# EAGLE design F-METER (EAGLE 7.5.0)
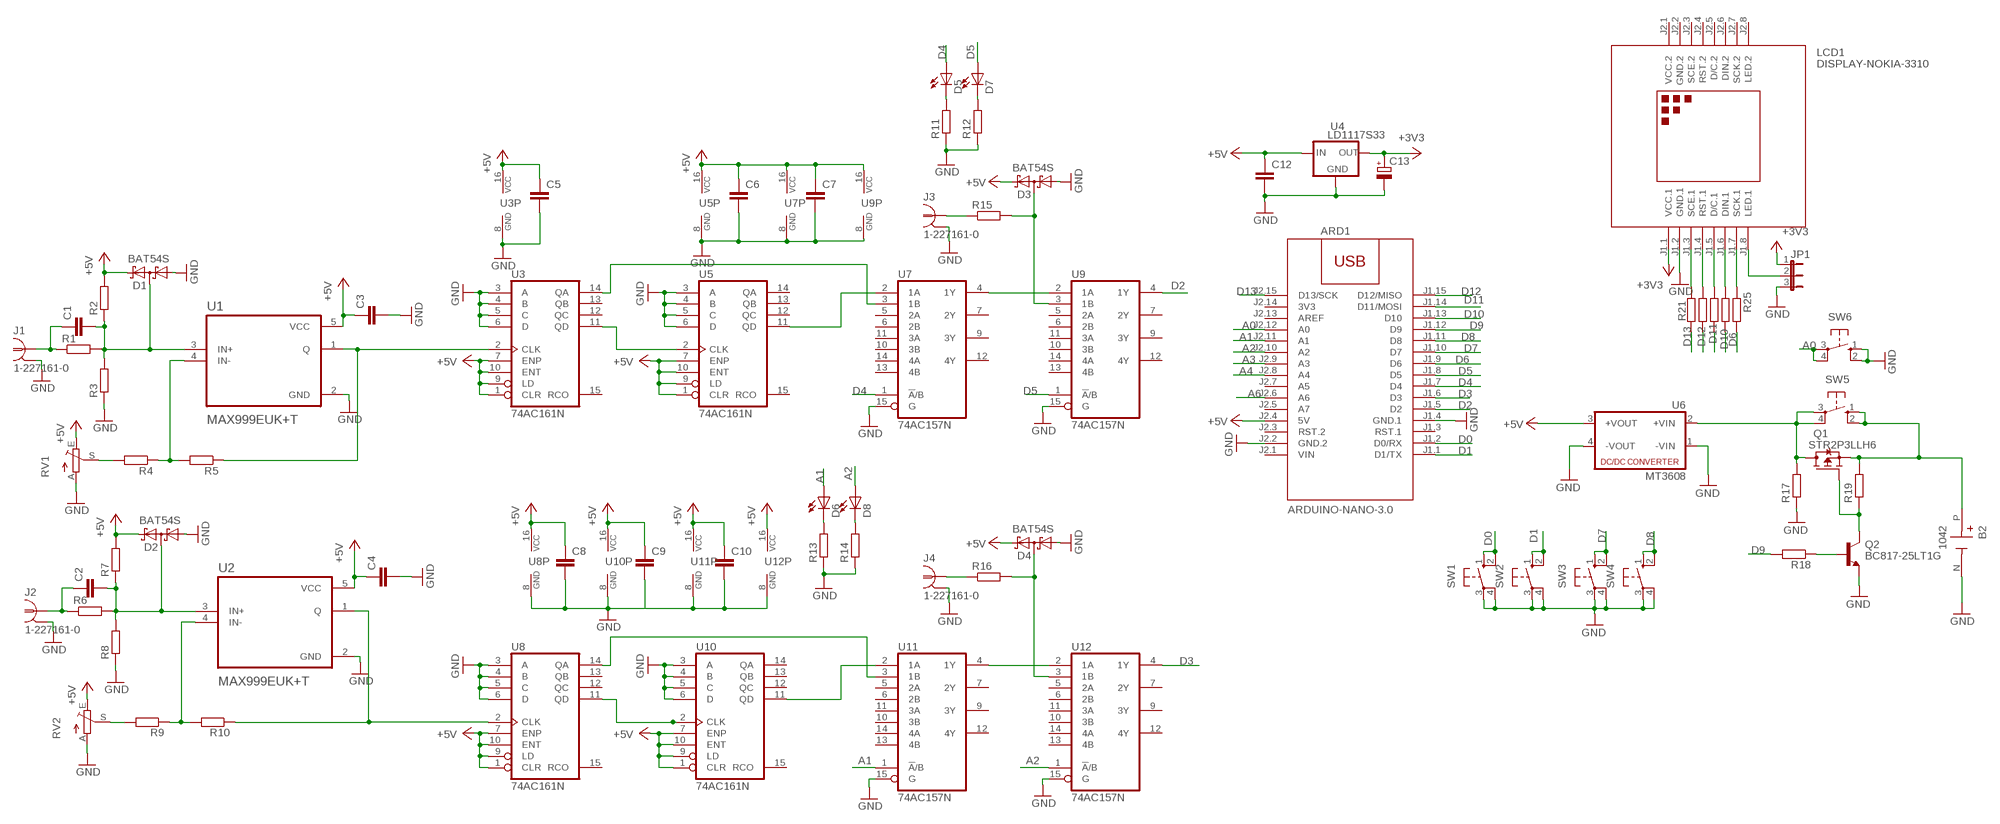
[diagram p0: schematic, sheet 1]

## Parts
ARD1  ARDUINO-NANO-3.0  [ARDUINO-NANO-3.0]
B2  1042  [BAT_1042]
C1  C-EUC1206  [C1206]
C2  C-EUC1206  [C1206]
C3  C-EUC1206  [C1206]
C4  C-EUC1206  [C1206]
C5  C-EUC1206  [C1206]
C6  C-EUC1206  [C1206]
C7  C-EUC1206  [C1206]
C8  C-EUC1206  [C1206]
C9  C-EUC1206  [C1206]
C10  C-EUC1206  [C1206]
C12  C-EUC1206  [C1206]
C13  CPOL-EUSMCD  [SMC_D]
D1  BAT54S  [SOT23]
D2  BAT54S  [SOT23]
D3  BAT54S  [SOT23]
D4  BAT54S  [SOT23]
D5  LED3MM  [LED3MM]
D6  LED3MM  [LED3MM]
D7  LED3MM  [LED3MM]
D8  LED3MM  [LED3MM]
J1  1-227161-0  [AMP_227161]
J2  1-227161-0  [AMP_227161]
J3  1-227161-0  [AMP_227161]
J4  1-227161-0  [AMP_227161]
JP1  JP2E  [JP2]
LCD1  DISPLAY-NOKIA-3310  [DISPLAY-NOKIA-3310]
Q1  STR2P3LLH6  [SOT23]
Q2  BC817-25LT1G  [SOT95P237X111-3N]
R1  R-EU_R1206  [R1206]
R2  R-EU_R1206  [R1206]
R3  R-EU_R1206  [R1206]
R4  R-EU_R1206  [R1206]
R5  R-EU_R1206  [R1206]
R6  R-EU_R1206  [R1206]
R7  R-EU_R1206  [R1206]
R8  R-EU_R1206  [R1206]
R9  R-EU_R1206  [R1206]
R10  R-EU_R1206  [R1206]
R11  R-EU_R1206  [R1206]
R12  R-EU_R1206  [R1206]
R13  R-EU_R1206  [R1206]
R14  R-EU_R1206  [R1206]
R15  R-EU_R1206  [R1206]
R16  R-EU_R1206  [R1206]
R17  R-EU_R1206  [R1206]
R18  R-EU_R1206  [R1206]
R19  R-EU_R1206  [R1206]
R21  R-EU_R1206  [R1206]
R22  R-EU_R1206  [R1206]
R23  R-EU_R1206  [R1206]
R24  R-EU_R1206  [R1206]
R25  R-EU_R1206  [R1206]
RV1  TRIM_EU-B64W  [B64W]
RV2  TRIM_EU-B64W  [B64W]
SW1  10-XX  [B3F-10XX]
SW2  10-XX  [B3F-10XX]
SW3  10-XX  [B3F-10XX]
SW4  10-XX  [B3F-10XX]
SW5  10-XX  [B3F-10XX]
SW6  10-XX  [B3F-10XX]
U1  MAX999EUK+T  [SOT95P280X145-5N]
U2  MAX999EUK+T  [SOT95P280X145-5N]
U3  74AC161N  74AC160N  [DIL16]
U4  LD1117S33  LD1117  [SOT223]
U5  74AC161N  74AC160N  [DIL16]
U6  MT3608  [MT3608]
U7  74AC157N  [DIL16]
U8  74AC161N  74AC160N  [DIL16]
U9  74AC157N  [DIL16]
U10  74AC161N  74AC160N  [DIL16]
U11  74AC157N  [DIL16]
U12  74AC157N  [DIL16]

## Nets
+3V3: C13.+ JP1.1 LCD1.J1.1(VCC.1) U4.2(OUT)
+5V: ARD1.J2.4(5V) C3.1 C4.1 C5.1 C6.1 C7.1 C8.1 C9.1 C10.1 C12.1 D1.2(C2) D2.2(C2) D3.2(C2) D4.2(C2) R2.2 R7.2 RV1.E RV2.E U1.5(VCC) U2.5(VCC) U3.1(CLR) U3.7(ENP) U3.9(LD) U3.10(ENT) U3.16(VCC) U4.3(IN) U5.1(CLR) U5.7(ENP) U5.9(LD) U5.10(ENT) U5.16(VCC) U6.3(+VOUT) U7.16(VCC) U8.1(CLR) U8.7(ENP) U8.9(LD) U8.10(ENT) U8.16(VCC) U9.16(VCC) U10.1(CLR) U10.7(ENP) U10.9(LD) U10.10(ENT) U10.16(VCC) U11.16(VCC) U12.16(VCC)
A0: ARD1.J2.12(A0) SW6.3(P) SW6.4(P1)
A1: ARD1.J2.11(A1) D6.A U11.1(!A!/B)
A2: ARD1.J2.10(A2) D8.A U12.1(!A!/B)
A3: ARD1.J2.9(A3)
A4: ARD1.J2.8(A4)
A6: ARD1.J2.6(A6)
D0: ARD1.J1.2(D0/RX) SW1.1(S) SW1.2(S1)
D1: ARD1.J1.1(D1/TX) SW2.1(S) SW2.2(S1)
D2: ARD1.J1.5(D2) U9.4(1Y)
D3: ARD1.J1.6(D3) U12.4(1Y)
D4: ARD1.J1.7(D4) D5.A U7.1(!A!/B)
D5: ARD1.J1.8(D5) D7.A U9.1(!A!/B)
D6: ARD1.J1.9(D6) R25.2
D7: ARD1.J1.10(D7) SW3.1(S) SW3.2(S1)
D8: ARD1.J1.11(D8) SW4.1(S) SW4.2(S1)
D9: ARD1.J1.12(D9) R18.2
D10: ARD1.J1.13(D10) R24.2
D11: ARD1.J1.14(D11/MOSI) R23.2
D12: ARD1.J1.15(D12/MISO) R22.2
D13: ARD1.J2.15(D13/SCK) R21.2
GND: ARD1.J1.4(GND.1) ARD1.J2.2(GND.2) B2.N(NEG) C3.2 C4.2 C5.2 C6.2 C7.2 C8.2 C9.2 C10.2 C12.2 C13.- D1.1(A1) D2.1(A1) D3.1(A1) D4.1(A1) J1.2 J2.2 J3.2 J4.2 JP1.3 LCD1.J1.2(GND.1) Q2.2(E) R3.1 R8.1 R11.1 R12.1 R13.1 R14.1 R17.1 RV1.A RV2.A SW1.3(P) SW1.4(P1) SW2.3(P) SW2.4(P1) SW3.3(P) SW3.4(P1) SW4.3(P) SW4.4(P1) SW6.1(S) SW6.2(S1) U1.2(GND) U2.2(GND) U3.3(A) U3.4(B) U3.5(C) U3.6(D) U3.8(GND) U4.1(GND) U5.3(A) U5.4(B) U5.5(C) U5.6(D) U5.8(GND) U6.1(-VIN) U6.4(-VOUT) U7.8(GND) U7.15(G) U8.3(A) U8.4(B) U8.5(C) U8.6(D) U8.8(GND) U9.8(GND) U9.15(G) U10.3(A) U10.4(B) U10.5(C) U10.6(D) U10.8(GND) U11.8(GND) U11.15(G) U12.8(GND) U12.15(G)
N$1: C1.1 J1.1 R1.1
N$2: C1.2 D1.3(C1A2) R1.2 R2.1 R3.2 U1.3(IN+)
N$3: R4.2 RV1.S
N$4: R4.1 R5.2 U1.4(IN-)
N$5: R5.1 U1.1(Q) U3.2(CLK)
N$6: C2.1 J2.1 R6.1
N$7: C2.2 D2.3(C1A2) R6.2 R7.1 R8.2 U2.3(IN+)
N$8: R9.1 R10.2 U2.4(IN-)
N$9: R9.2 RV2.S
N$10: R10.1 U2.1(Q) U8.2(CLK)
N$11: U3.11(QD) U5.2(CLK)
N$12: U5.11(QD) U7.2(1A)
N$13: U3.14(QA) U7.3(1B)
N$14: U7.4(1Y) U9.2(1A)
N$15: J3.1 R15.1
N$16: D3.3(C1A2) R15.2 U9.3(1B)
N$17: Q1.2(G) Q2.3(C) R19.1
N$18: LCD1.J1.3(SCE.1) R21.1
N$19: LCD1.J1.4(RST.1) R22.1
N$20: LCD1.J1.5(D/C.1) R23.1
N$21: LCD1.J1.6(DIN.1) R24.1
N$22: LCD1.J1.7(SCK.1) R25.1
N$23: B2.P(POS) Q1.3(S) R19.2 SW5.1(S) SW5.2(S1)
N$24: Q2.1(B) R18.1
N$26: Q1.1(D) R17.2 SW5.3(P) SW5.4(P1) U6.2(+VIN)
N$28: JP1.2 LCD1.J1.8(LED.1)
N$29: D5.K(C) R11.2
N$30: D7.K(C) R12.2
N$31: J4.1 R16.1
N$32: D4.3(C1A2) R16.2 U12.3(1B)
N$33: U8.11(QD) U10.2(CLK)
N$34: U10.11(QD) U11.2(1A)
N$35: U8.14(QA) U11.3(1B)
N$36: U11.4(1Y) U12.2(1A)
N$39: D6.K(C) R13.2
N$40: D8.K(C) R14.2
Unconnected: ARD1.J1.3(RST.1) ARD1.J2.3(RST.2) ARD1.J2.5(A7) ARD1.J2.7(A5) ARD1.J2.13(AREF) LCD1.J2.3(SCE.2) LCD1.J2.4(RST.2) LCD1.J2.5(D/C.2) LCD1.J2.6(DIN.2) LCD1.J2.7(SCK.2) LCD1.J2.8(LED.2) U3.12(QC) U3.13(QB) U3.15(RCO) U5.12(QC) U5.13(QB) U5.14(QA) U5.15(RCO) U7.5(2A) U7.6(2B) U7.7(2Y) U7.9(3Y) U7.10(3B) U7.11(3A) U7.12(4Y) U7.13(4B) U7.14(4A) U8.12(QC) U8.13(QB) U8.15(RCO) U9.5(2A) U9.6(2B) U9.7(2Y) U9.9(3Y) U9.10(3B) U9.11(3A) U9.12(4Y) U9.13(4B) U9.14(4A) U10.12(QC) U10.13(QB) U10.14(QA) U10.15(RCO) U11.5(2A) U11.6(2B) U11.7(2Y) U11.9(3Y) U11.10(3B) U11.11(3A) U11.12(4Y) U11.13(4B) U11.14(4A) U12.5(2A) U12.6(2B) U12.7(2Y) U12.9(3Y) U12.10(3B) U12.11(3A) U12.12(4Y) U12.13(4B) U12.14(4A)

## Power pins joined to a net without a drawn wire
3V3: ARD1.J2.14(3V3)
GND.2: LCD1.J2.2(GND.2)
VCC.2: LCD1.J2.1(VCC.2)
VIN: ARD1.J2.1(VIN)

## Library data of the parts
ARD1 = diy-modules:ARDUINO-NANO-3.0: Arduino Nano 3.0 and compatible devices More details available here: https://www.arduino.cc/en/Main/ArduinoBoardNano Click here to find device on ebay.com
B2 = 18650-HOLDER:1042: Check availability; AVAILABILITY: In Stock; CHECK_PRICES: https://www.snapeda.com/parts/1042/Keystone/view-part/?ref=eda; DESCRIPTION: SMT Holder for 18650 Battery; MF: Keystone Electronics Corp.; MP: 1042; PACKAGE: NON STANDARD-5 Keystone; PRICE: None; SNAPEDA_LINK: https://www.snapeda.com/parts/1042/Keystone/view-part/?ref=snap
C1-C10 C12 = rcl:C-EU: CAPACITOR, European symbol
C13 = rcl:CPOL-EU: POLARIZED CAPACITOR, European symbol
D1-D4 = diode:BAT54S: Schottky Diodes Pin connection corrected 2011-05-04 Source: Fairchild .. BAT54.pdf
D5-D8 = led:LED: LED
J1-J4 = con-coax:?227161*: JACK, RIGHT ANGLE, 50 OHM, PCB, BNC; MF: TYCO ELECTRONICS; MPN: 1-227161; OC_FARNELL: unknown; OC_NEWARK: 33B3200
JP1 = jumper:JP2E: JUMPER
LCD1 = diy-modules:DISPLAY-NOKIA-3310: 84x48 Dot Matrix LCD Module based on Nokia 3310 display More details available here: https://arduinoandsoftware.wordpress.com/2012/12/30/nokia-33105110-3-3v-display-with-5v-arduino/
Q1 = transistor-fet:STR2P3LLH6
Q2 = BC817-25LT1G:BC817-25LT1G: Check availability; AVAILABILITY: In Stock; CHECK_PRICES: https://www.snapeda.com/parts/BC817-25LT1G/Onsemi/view-part/?ref=eda; DESCRIPTION: Transistor NPN 45V 0.5A hfe160 SOT23 | ON Semiconductor BC817-25LT1G; MF: ON Semiconductor; MP: BC817-25LT1G; PACKAGE: SOT-23-3 ON Semiconductor; PRICE: None; PURCHASE-URL: https://www.snapeda.com/api/url_track_click_mouser/?unipart_id=343725&manufacturer=ON Semiconductor&part_name=BC817-25LT1G&search_term=transistor sot23; SNAPEDA_LINK: https://www.snapeda.com/parts/BC817-25LT1G/Onsemi/view-part/?ref=snap
R1-R19 R21-R25 = rcl:R-EU_: RESISTOR, European symbol
RV1 RV2 = pot:TRIM_EU-: POTENTIOMETER
SW1-SW6 = switch-omron:10-XX: OMRON SWITCH; MPN: B3F-1000; OC_FARNELL: 176432; OC_NEWARK: 36M3542
U1 U2 = MAX999EUK_T:MAX999EUK+T: Check availability; AVAILABILITY: In Stock; CHECK_PRICES: https://www.snapeda.com/parts/MAX999EUK+T/Analog+Devices/view-part/?ref=eda; DESCRIPTION: Single/Dual/Quad, Ultra-High-Speed, +3V/+5V, Beyond-the-Rails Comparators; MF: Analog Devices; MP: MAX999EUK+T; PACKAGE: SOT-23-5 Maxim Integrated; PRICE: None; SNAPEDA_LINK: https://www.snapeda.com/parts/MAX999EUK+T/Analog+Devices/view-part/?ref=snap
U3 U5 U8 U10 = 74xx-eu:74*160: Synchronous 4-bit COUNTER
U4 = v-reg:LD1117
U6 = dc-dc-converter:MT3608: DC DC Up Converter
U7 U9 U11 U12 = 74xx-eu:74*157: Quadruple 2-line to 1-line data SELECTOR/MULTIPLEXER

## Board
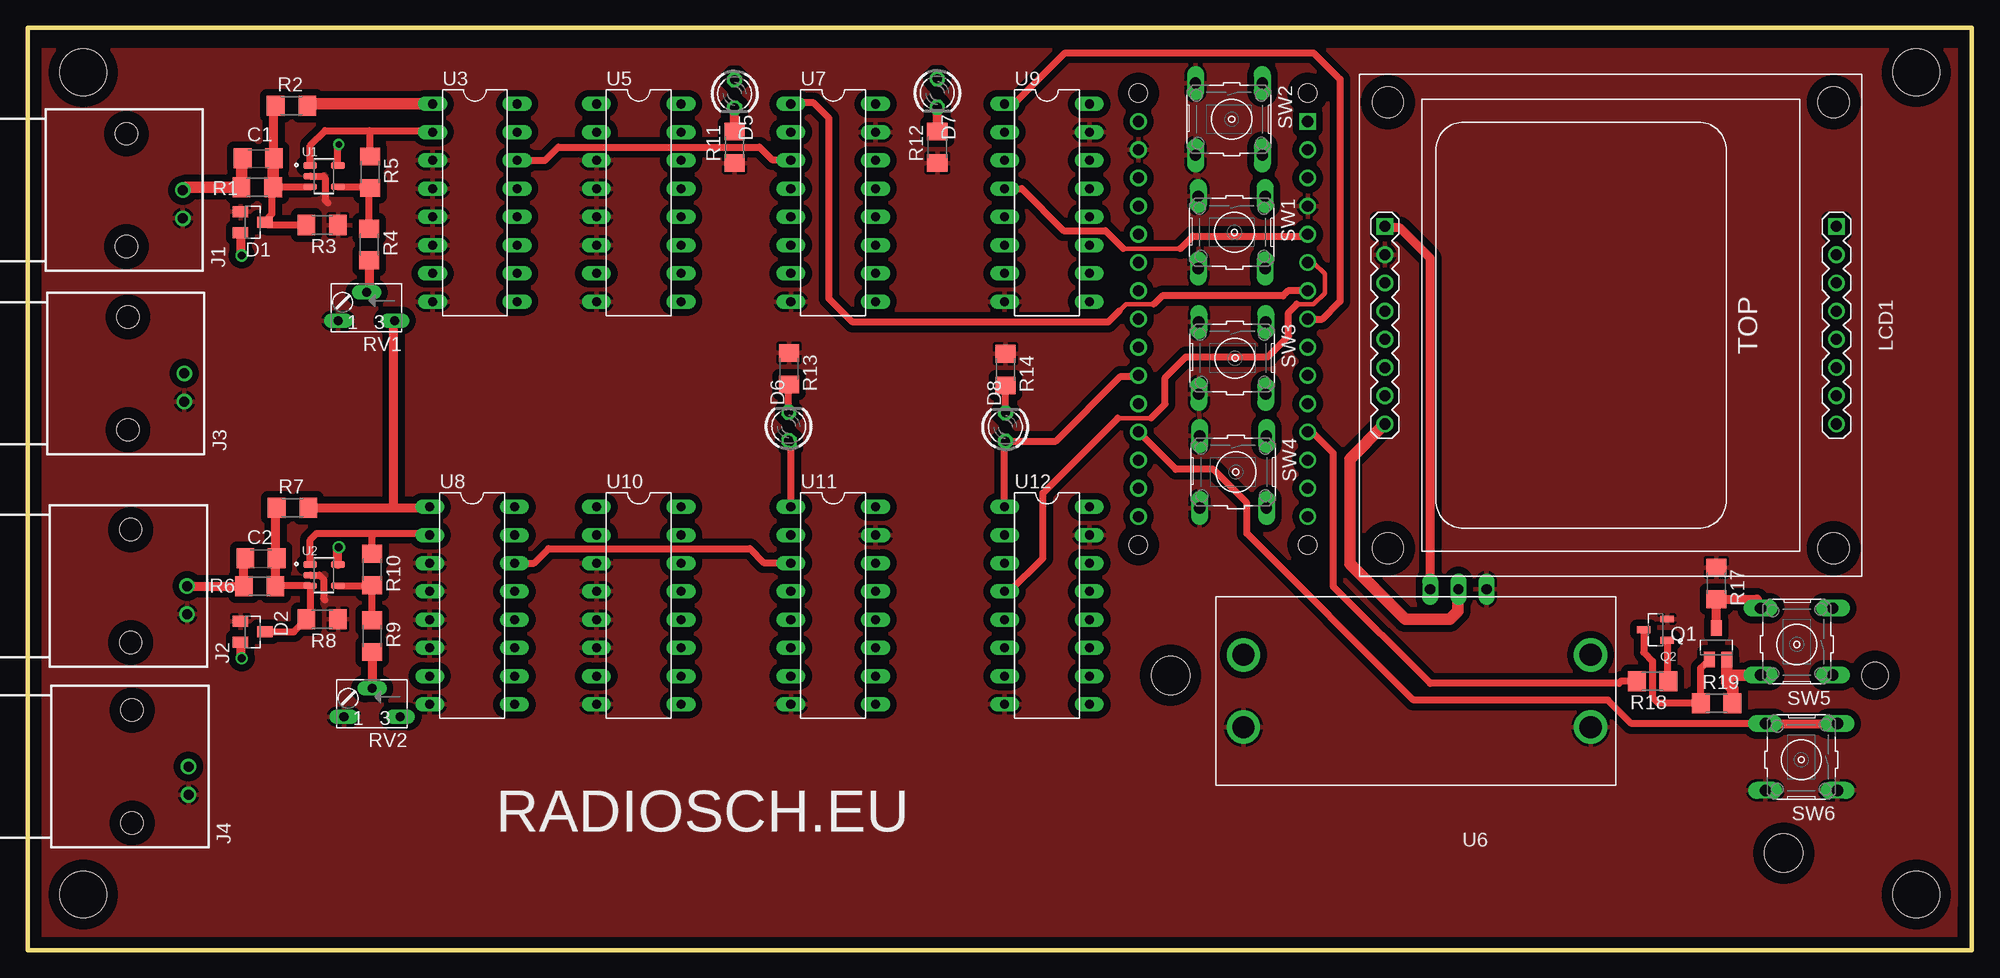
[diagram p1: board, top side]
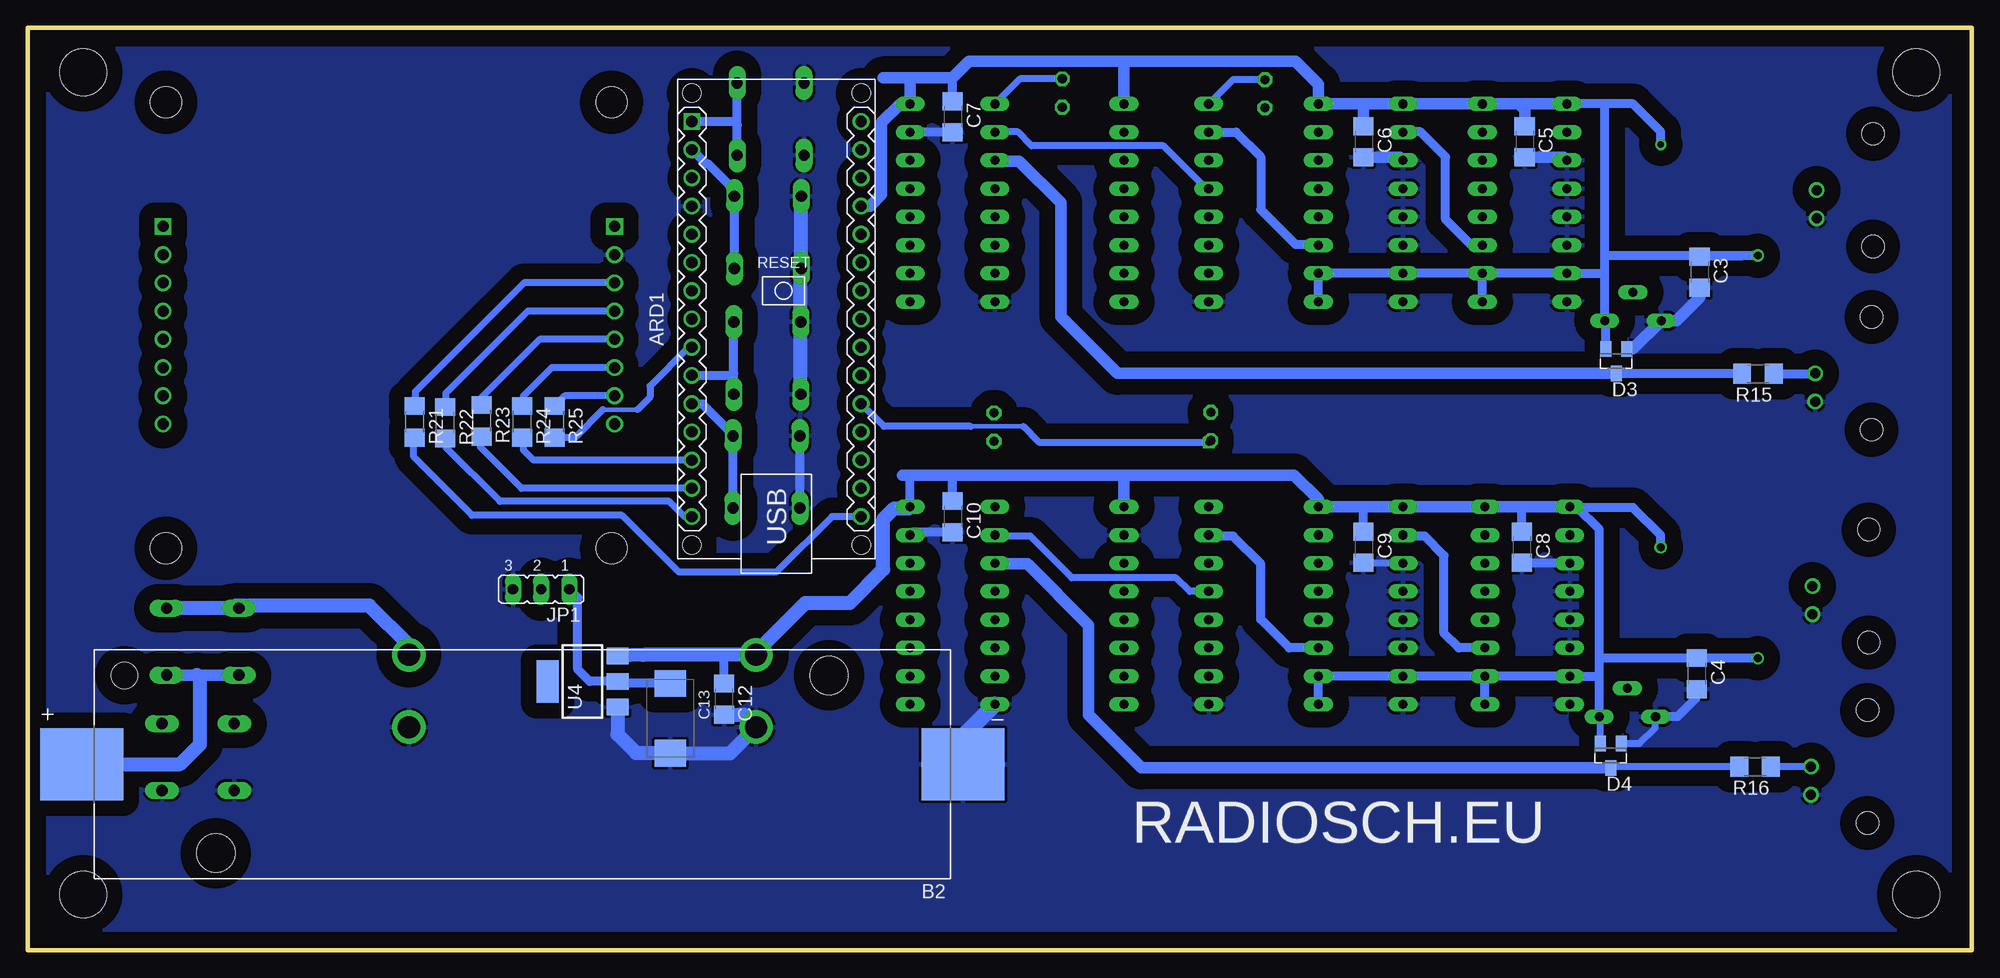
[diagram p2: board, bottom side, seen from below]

Size 175 x 83 mm. Coordinates in mm from the lower left corner, seen from the top.
Outline: 0,0 175,0 175,83 0,83 0,0
Copper layers (1*16): Top 0.035mm / dielectric 1.5mm / Bottom 0.035mm
Design rules "default": minimum track width 10mil, minimum drill 24mil, track to track 8mil, track to pad 8mil, pad to pad 8mil, via to via 8mil, smd to smd 8mil, copper to edge 40mil, drill to drill 8mil, minimum pad ring 10mil, minimum via ring 8mil, stop-mask expansion 4mil, vias tented up to drill 0mil, thermal gap 10mil
Holes 4.2 mm at 5,79 5,5 170,5 170,79

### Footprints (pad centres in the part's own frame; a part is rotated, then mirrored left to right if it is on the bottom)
ARDUINO-NANO-3.0 = drill 1 square: J1.1 17.78,7.62 | drill 1: J1.2 15.24,7.62; J1.3 12.7,7.62; J1.4 10.16,7.62; J1.5 7.62,7.62; J1.6 5.08,7.62; J1.7 2.54,7.62; J1.8 0,7.62; J1.9 -2.54,7.62; J1.10 -5.08,7.62; J1.11 -7.62,7.62; J1.12 -10.16,7.62; J1.13 -12.7,7.62; J1.14 -15.24,7.62; J1.15 -17.78,7.62; J2.1 17.78,-7.62; J2.2 15.24,-7.62; J2.3 12.7,-7.62; J2.4 10.16,-7.62; J2.5 7.62,-7.62; J2.6 5.08,-7.62; J2.7 2.54,-7.62; J2.8 0,-7.62; J2.9 -2.54,-7.62; J2.10 -5.08,-7.62; J2.11 -7.62,-7.62; J2.12 -10.16,-7.62; J2.13 -12.7,-7.62; J2.14 -15.24,-7.62; J2.15 -17.78,-7.62 | hole 1.651: -20.32,7.62; -20.32,-7.62; 20.32,-7.62; 20.32,7.62
BAT_1042 = smd 7.46 x 6.47: N -39.67,0; P 39.67,0 | hole 3.45: 27.6,8; -27.6,-8 | hole 2.39: 35.82,-8
C1206 = smd 1.6 x 1.8: 1 -1.4,0; 2 1.4,0
SMC_D = smd 2.4 x 2.8: + -3.15,0; - 3.15,0
SOT23 = smd 1 x 1.4: 1 -0.95,-1.1; 2 0.95,-1.1; 3 0,1.1
LED3MM = drill 0.813 octagon: A -1.27,0; K 1.27,0
AMP_227161 = drill 0.9 pad 1.27: 1 0,-5.08; 2 -2.54,-5.08 | hole 2: -5.08,0; 5.08,0
JP2 = drill 0.914 long: 1 -2.54,0; 2 0,0; 3 2.54,0
DISPLAY-NOKIA-3310 = drill 1 square: J1.1 -8.89,-20.32; J2.1 -8.89,20.32 | drill 1: J1.2 -6.35,-20.32; J1.3 -3.81,-20.32; J1.4 -1.27,-20.32; J1.5 1.27,-20.32; J1.6 3.81,-20.32; J1.7 6.35,-20.32; J1.8 8.89,-20.32; J2.2 -6.35,20.32; J2.3 -3.81,20.32; J2.4 -1.27,20.32; J2.5 1.27,20.32; J2.6 3.81,20.32; J2.7 6.35,20.32; J2.8 8.89,20.32 | hole 2.8: -20.066,-20.066; 20.066,-20.066; 20.066,20.066; -20.066,20.066
SOT23' = smd 1 x 1.4: 1 0,1.735; 2 -0.632,-1.1; 3 0.95,-1.1
SOT95P237X111-3N = smd 1.23 x 0.6: 1 -1.06,0.95; 2 -1.06,-0.95; 3 1.06,0
R1206 = smd 1.6 x 1.803: 1 -1.422,0; 2 1.422,0
B64W = drill 0.813 long: A 2.54,0; E -2.54,0; S 0,-2.54
B3F-10XX = drill 1.016 long: 1 -3.251,2.761; 2 3.251,2.761; 3 -3.251,-3.261; 4 3.251,-3.261
SOT95P280X145-5N = smd 1.22 x 0.6: 1 -1.245,0.95; 2 -1.245,0; 3 -1.245,-0.95; 4 1.245,-0.95; 5 1.245,0.95
DIL16 = drill 0.813 long: 1 -8.89,-3.81; 2 -6.35,-3.81; 3 -3.81,-3.81; 4 -1.27,-3.81; 5 1.27,-3.81; 6 3.81,-3.81; 7 6.35,-3.81; 8 8.89,-3.81; 9 8.89,3.81; 10 6.35,3.81; 11 3.81,3.81; 12 1.27,3.81; 13 -1.27,3.81; 14 -3.81,3.81; 15 -6.35,3.81; 16 -8.89,3.81
SOT223 = smd 1.5 x 2: 1 -2.3,-3.15; 2 0,-3.15; 3 2.3,-3.15 | smd 3.8 x 2: 4 0,3.15
MT3608 = drill 2: 1 2.25,11.75; 2 2.25,5.25; 3 33.5,5.25; 4 33.5,11.75

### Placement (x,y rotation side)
ARD1  107.6,56.79 90 bottom
B2  130.47,16.72 180 bottom
C1  20.75,71.25 0 top
C2  21,35.25 0 top
C3  24.5,61 270 bottom
C4  24.75,24.88 270 bottom
C5  40.25,72.75 270 bottom
C6  54.75,72.75 270 bottom
C7  91.75,75 270 bottom
C8  40.5,36.25 270 bottom
C9  54.75,36.25 270 bottom
C10  91.75,39 270 bottom
C12  112.33,22.58 270 bottom
C13  117.16,20.85 270 bottom
D1  20.25,65.5 270 top
D2  20.25,28.63 270 top
D3  32,53 180 bottom
D4  32.5,17.5 180 bottom
D5  63.63,77.06 270 top
D6  68.5,47.12 90 top
D7  81.88,77.12 270 top
D8  88.01,47.06 90 top
J1  8.89,68.39 90 top
J2  9.27,32.76 90 top
J3  9.02,51.9 90 top
J4  9.39,16.51 90 top
JP1  128.79,32.46 180 bottom
LCD1  142.5,56.23 270 top
Q1  STR2P3LLH6  [SOT23']  152.01,27.23 0 top
Q2  146.52,28.83 180 top
R1  20.66,68.66 0 top
R2  23.75,76 0 top
R3  26.5,65.25 180 top
R4  30.75,63.5 270 top
R5  30.81,70 270 top
R6  20.88,32.75 0 top
R7  23.84,39.81 0 top
R8  26.5,29.75 180 top
R9  31,28.25 270 top
R10  31,34.25 270 top
R11  63.62,72.25 90 top
R12  81.88,72.25 90 top
R13  68.52,52.31 270 top
R14  88.02,52.23 270 top
R15  19.25,51.88 180 bottom
R16  19.5,16.5 180 bottom
R17  152,33 270 top
R18  146.27,24.2 180 top
R19  152.03,22.21 0 top
R21  140.16,47.53 270 bottom
R22  137.41,47.45 270 bottom
R23  134.16,47.62 270 bottom
R24  130.5,47.53 270 bottom
R25  127.58,47.53 270 bottom
RV1  30.5,56.64 180 top
RV2  31,21 180 top
SW1  108.63,64.59 270 top
SW2  108.38,74.77 270 top
SW3  108.68,53.27 270 top
SW4  108.75,43.02 270 top
SW5  159.25,27.5 180 top
SW6  159.66,17.12 180 top
U1  26.67,69.64 0 top
U2  26.67,33.73 0 top
U3  40.25,67.25 270 top
U4  125.06,24.17 90 bottom
U5  55,67.25 270 top
U6  142.94,31.81 180 top
U7  72.5,67.25 270 top
U8  40,31 270 top
U9  91.75,67.25 270 top
U10  55,31 270 top
U11  72.5,31 270 top
U12  91.75,31 270 top

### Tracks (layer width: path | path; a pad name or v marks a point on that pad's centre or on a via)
+3V3
  Top 0.813: JP1.1 126.25,62.25 123.5,65 122.3,65 LCD1.J1.1
  Bottom 0.813: C13.+ 121.74,24 U4.2 124.42,24.17 125.5,25.25 125.5,31.71 JP1.1
+5V  (via drill 0.6, 0.7)
  Top 0.61: U1.5 27.91,72.42 v28,72.5
  Top 0.813: D1.2 19.15,62.6 v19.25,62.5 | R7.2 32.75,39.81 | 32.75,39.81 36.11,39.81 U8.1 | U2.5 27.91,36.16 v28,36.25 | D2.2 19.15,26.35 v19.25,26.25 | 32.75,39.81 32.95,40.01 32.95,56.55 RV1.E
  Top 1.016: U3.1 25.31,76.14 R2.2
  Bottom 0.61: C3.1 20.6,62.4 20.5,62.5 | D4.2 33.45,20.91 RV2.E
  Bottom 0.813: v28,72.5 28,73.64 30.5,76.14 33.25,76.14 | 33.25,76.14 U3.1 | RV1.E 33.04,60.75 | 33.04,60.75 33.04,62.5 | 33.04,62.5 33.04,75.93 33.25,76.14 | 33.04,60.75 33.19,60.9 U3.7 U3.10 44.62,60.9 | v19.25,62.5 20.5,62.5 33.04,62.5 | 44.62,60.9 U5.7 U5.10 U5.9 | U3.9 44.06,60.33 44.62,60.9 | v28,36.25 28,37.31 30.5,39.81 35.5,39.81 | 35.5,39.81 36.11,39.81 U8.1 | v19.25,26.25 24.73,26.25 C4.1 33.31,26.27 33.54,26.5 | RV2.E 33.54,24.5 | 33.54,24.5 33.54,26.5 | 33.54,26.5 33.54,37.85 35.5,39.81 | D3.2 32.95,56.55 | 33.54,24.5 33.69,24.65 U8.7 U8.10 | U12.16 95.56,42.56 95.75,42.75 | C8.1 40.5,39.64 40.75,39.89 | C7.1 91.75,78.5 | C10.1 91.75,42.75 | C9.1 54.75,39.64 54.5,39.89 | U8.10 U10.7 U10.10 U10.9 | U8.9 U8.10 | C12.1 112.33,26.39 112.5,26.56
  Bottom 1.016: U3.1 40.75,76.14 | 40.75,76.14 U3.16 U5.1 54.5,76.14 | 54.5,76.14 U5.16 | C5.1 40.25,75.64 40.75,76.14 | U5.16 58.81,76.31 | 95.5,78.5 91.75,78.5 90.25,80 76.5,80 | 95.5,78.5 98,78.5 | 95.5,78.5 95.56,78.44 U9.16 95.58,76.12 96.5,76.12 98.12,74.5 98.12,68 99.17,66.95 ARD1.J2.4 | C6.1 54.75,75.89 54.5,76.14 | U8.1 40.75,39.89 U8.16 U10.1 54.5,39.89 U10.16 58.81,40.56 61,42.75 76,42.75 | 76,42.75 91.75,42.75 95.75,42.75 96.25,42.75 | U11.16 76.31,42.44 76,42.75 | 32.95,56.55 RV1.E | U5.16 58.81,77.94 60.88,80 76.5,80 | U7.16 76.31,79.81 76.5,80
  Bottom 1.27: U12.16 95.7,39.75 97,39.75 98,38.75 98,34.25 101,31.25 105,31.25 109.44,26.81 U6.3 112.5,26.56 119.57,26.56 U4.3
A0
  Top 0.61: SW6.4 144.37,20.38 142.25,22.5 124.75,22.5 109.75,37.5 109.75,40.25 106.75,43.25 103.36,43.25 ARD1.J2.12
  Top 0.813: SW6.4 SW6.3
A1  (via drill 0.6)
  Top 0.61: U11.1 v68.69,45.66 D6.A
  Bottom 0.406: 85.38,47.12 90.12,47.12
  Bottom 0.61: v68.69,45.66 83.92,45.66 85.38,47.12 | 90.12,47.12 97.94,47.12 ARD1.J2.11
A2
  Top 0.61: U12.1 87.94,45.73 D8.A 92.55,45.8 98.38,51.62 99.89,51.62 ARD1.J2.10
D0
  Bottom 0.813: SW1.2 SW1.1 111.39,68.39 113.75,70.75 113.94,70.75 ARD1.J1.2
D1
  Bottom 0.813: SW2.2 111.14,74.25 | 111.14,74.25 SW2.1 | ARD1.J1.1 111.46,74.57 111.14,74.25
D2
  Top 0.406: 98.62,63.12 103.75,63.12
  Top 0.61: U9.4 89.48,68.52 93.25,64.75 97,64.75 98.62,63.12 | 103.75,63.12 104.88,64.25 115.06,64.25 ARD1.J1.5
D3
  Top 0.406: 98.12,47.88 101.12,47.88 | 114.25,58.12 115.75,58.12 116.75,59.12 116.75,60.88 115.75,61.88 ARD1.J1.6
  Top 0.61: U12.4 88.39,32.27 91.38,35.25 91.38,41.12 98.12,47.88 | 101.12,47.88 102.38,49.12 102.38,51.5 104.25,53.38 111.62,53.38 113.5,55.25 113.5,57.38 114.25,58.12
D4
  Top 0.406: 101.38,58.12 98.88,58.12 98.25,57.5
  Top 0.61: ARD1.J1.7 113.45,59.33 113,58.88 102.12,58.88 101.38,58.12 | 98.25,57.5 97.25,56.5 74.25,56.5 72.12,58.62 72.12,74.88 70.75,76.25 68.8,76.25 U7.1
  Bottom 0.61: D5.A 66.5,78.33 U7.1
D5
  Top 0.61: U9.1 88.77,76.14 93.38,80.75 115.75,80.75 118.12,78.38 118.12,58.38 116.54,56.79 ARD1.J1.8
  Bottom 0.61: D7.A 85.69,78.39 U9.1
D6
  Bottom 0.406: 120.12,48.62 123.25,48.62
  Bottom 0.61: ARD1.J1.9 115.5,54.25 119,50.75 119,49.75 120.12,48.62 | 123.25,48.62 125.75,46.12 127.56,46.12 R25.2
D7
  Bottom 0.813: SW3.2 111.44,51.88 | 111.44,51.88 SW3.1 | ARD1.J1.10 111.61,51.71 111.44,51.88
D8
  Bottom 0.813: SW4.2 SW4.1 111.51,46.39 114.25,49.12 115.17,49.12 ARD1.J1.11
D9
  Top 0.61: R18.2 143.45,24.2 143.25,24 126.25,24 117.5,32.75 117.5,44.75 115.62,46.63 ARD1.J1.12
D10
  Bottom 0.61: ARD1.J1.13 129.47,44.09 130.38,45 130.38,45.98 R24.2
D11
  Bottom 0.61: ARD1.J1.14 130.55,41.55 134.25,45.25 134.25,46.11 R23.2
D12
  Bottom 0.61: R22.2 137.38,45.99 137.38,45.25 132.5,40.38 117.25,40.38 115.89,39.01 ARD1.J1.15
D13
  Bottom 0.61: ARD1.J2.15 102.61,39.01 107.62,34 116.38,34 121.5,39.12 135,39.12 140.25,44.38 140.25,46.02 R21.2
GND
  Top 0.61: U1.2 26.61,69.64 26.75,69.5 26.75,67.5 27,67.25 | U2.2 26.27,33.73 26.62,33.38 26.62,31.62 26.75,31.5
  Bottom 0.61: D4.1 29.9,18.6 28.5,20 28.5,20.96 RV2.A | C9.2 51.23,34.85 U10.3
  Bottom 0.813: C4.2 24.75,22.75 26.5,21 RV2.A | C8.2 36.23,34.85 U8.3 | C7.2 U9.15 | C10.2 95.31,37.6 U12.15 | SW4.4 SW4.3
  Bottom 1.016: C5.2 36.73,71.35 U3.3 | C3.2 24.5,58.75 26.61,56.64 RV1.A 30.5,54.1 D3.1 | C6.2 51.48,71.35 U5.3
  Bottom 1.27: C12.2 110.56,21.18 U6.4 111.8,17.7 C13.- 117.21,17.75 120.25,17.75 121.91,19.41 U4.1 | SW3.4 SW3.3 105.42,61.29 SW1.4 SW1.3
  Bottom 1.422: B2.N 90.8,19.25 U12.8
  pour Top (isolate 0.61): 1,81 174,81 173.5,0.25 0,0.25
  pour Bottom (isolate 1.422): 2,82 174,82 174,2 174,0 2,0
N$1
  Top 1.016: J1.1 14.24,68.66 R1.1 19.24,71.14 C1.1
N$2
  Top 0.61: U1.3 25.39,68.66 R1.2 22,68.58 22,66.25 21.35,65.6 D1.3 21.6,65.25 R3.2
  Top 0.813: C1.2 22.15,75.57 R2.1
  Top 1.016: R1.2 22.08,71.18 C1.2
N$3
  Top 0.813: R4.2 30.75,59.43 RV1.S
N$4
  Top 0.61: R4.1 30.75,68.52 R5.2 30.7,68.69 U1.4
N$5
  Top 0.61: U1.1 25.43,72.42 26.75,73.75 30.75,73.75 | 30.75,73.75 36.29,73.75 U3.2 | R5.1 30.81,73.69 30.75,73.75
N$6
  Top 0.813: C2.1 19.45,35.1 R6.1 J2.1
N$7
  Top 0.61: R6.2 22.33,32.78 U2.3 25.43,30.1 R8.2 23.96,28.63 D2.3
  Top 0.813: 22.33,35.18 22.33,39.72 R7.1 | 22.33,32.78 22.33,35.18 | 22.33,35.18 C2.2
N$8
  Top 0.61: U2.4 30.95,32.78 R10.2 R9.1
N$9
  Top 0.813: R9.2 RV2.S
N$10
  Top 0.61: U2.1 25.43,36.92 26,37.5 31.25,37.5 | 31.25,37.5 36.04,37.5 U8.2 | R10.1 31,37.25 31.25,37.5
N$11
  Bottom 0.813: U3.11 45.06,63.44 47.38,65.75 47.38,71.38 49.62,73.62 51.16,73.62 U5.2
N$12
  Bottom 0.813: U7.2 66.22,73.6 64,71.38 64,66.62 60.88,63.5 58.87,63.5 U5.11
N$13
  Top 0.61: U3.14 46.56,71.06 47.75,72.25 65.88,72.25 67,71.12 68.62,71.12 U7.3
N$14
  Bottom 0.61: U7.4 68.89,68.52 72.75,72.38 84.62,72.38 85.88,73.62 87.92,73.62 U9.2
N$15
  Bottom 0.813: R15.1 14.12,51.88 J3.1
N$16
  Bottom 0.813: R15.2 31.98,51.88 D3.3
  Bottom 1.016: D3.3 76.9,51.9 82,57 82,67.25 85.75,71 87.88,71 U9.3
N$17
  Top 0.61: Q2.3 145.46,26.79 146.25,26 146.25,22.75 146.75,22.25 150.57,22.25 R19.1 150.61,25.36 Q1.2
N$18
  Bottom 0.61: LCD1.J1.3 130.34,60.04 140.12,50.25 140.12,48.99 R21.1
N$19
  Bottom 0.61: LCD1.J1.4 130,57.5 137.38,50.12 137.38,48.91 R22.1
N$20
  Bottom 0.61: LCD1.J1.5 128.91,54.96 134.12,49.75 134.12,49.08 R23.1
N$21
  Bottom 0.61: LCD1.J1.6 127.83,52.42 130.38,49.88 130.38,49.08 R24.1
N$22
  Bottom 0.61: LCD1.J1.7 126.65,49.88 R25.1
N$23
  Top 1.016: Q1.3 152.96,24.75 | 152.96,24.75 152.96,24.04 153.5,23.5 153.5,22.26 R19.2 | SW5.2 152.97,24.74 152.96,24.75
  Bottom 1.016: SW5.2 159.75,24.74 SW5.1
  Bottom 1.27: B2.P 161.28,16.72 159.5,18.5 159.5,24.49 159.75,24.74
N$24
  Top 0.61: Q2.1 147.58,24.31 R18.1
N$26
  Top 0.813: Q1.1 152.01,31.57 R17.2 155.68,31.58 SW5.4
  Bottom 1.27: U6.2 140.69,27.44 144.25,31 156.26,31 SW5.4 SW5.3
N$28
  Top 1.016: LCD1.J1.8 119,44.16 119,34.75 124,29.75 128,29.75 128.75,30.5 128.75,32.42 JP1.2
N$29
  Top 0.813: R11.2 D5.K
N$30
  Top 0.813: R12.2 D7.K
N$31
  Bottom 0.61: J4.1 18.07,16.51 R16.1
N$32
  Bottom 0.61: R16.2 32.4,16.5 D4.3
  Bottom 1.016: D4.3 74.75,16.4 79.5,21.15 79.5,29.25 85,34.75 87.88,34.75 U12.3
N$33
  Bottom 0.813: U8.11 46.19,27.19 47.5,28.5 47.5,35.5 49.25,37.25 51.09,37.25 U10.2
N$34
  Bottom 0.813: U10.11 61.44,27.19 64,29.75 64,34.75 66.5,37.25 68.59,37.25 U11.2
N$35
  Top 0.61: U8.14 45.56,34.81 46.88,36.12 65,36.12 66.25,34.88 68.62,34.88 U11.3
N$36
  Bottom 0.61: U11.4 70.39,32.27 71.62,33.5 81,33.5 84.75,37.25 87.84,37.25 U12.2
N$39
  Top 0.61: D6.K 68.5,50.87 R13.2
N$40
  Top 0.61: D8.K R14.2

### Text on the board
tPlace: RADIOSCH.EU
bPlace: RADIOSCH.EU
